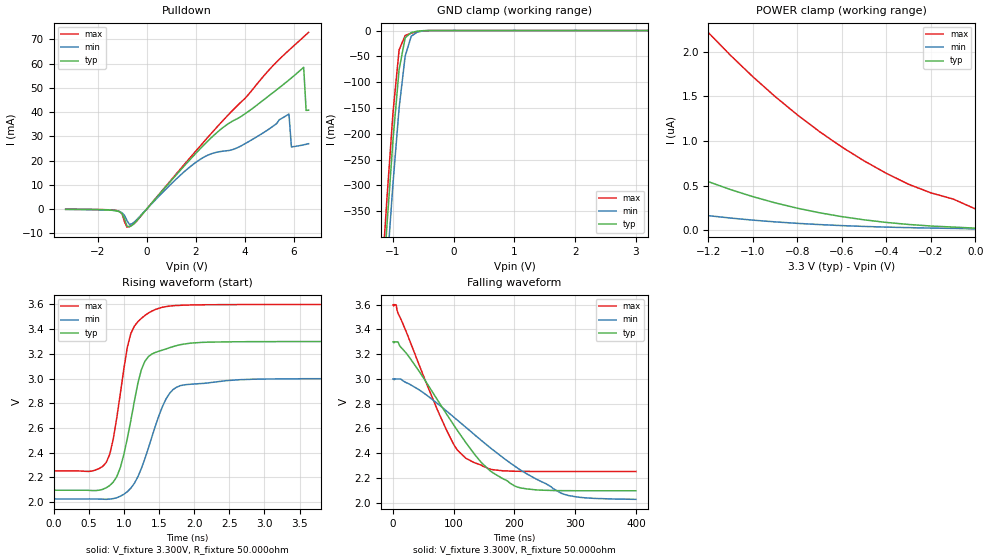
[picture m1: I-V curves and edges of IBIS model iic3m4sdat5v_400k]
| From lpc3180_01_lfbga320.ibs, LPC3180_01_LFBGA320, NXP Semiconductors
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| iic3m4sdat5v
|   IIC Pad
|   Serial Data Signal
| Normal 400 kHz Open-drain Mode (ehs=0)
[Model]   iic3m4sdat5v_400k | of iic3m4sdat5v
Model_type   I/O_open_drain
Polarity   Non-Inverting
|  Reciever Thresholds
Vinl   = 0.99V
Vinh   = 2.31V
| AC Test Load Conditions
Vref   = 0
Cref   = 0
Rref   = 1000000000
Vmeas   = 1.65
| [Process Range]   typical   min   max
| C_comp edge width   400.000ps   400.000ps   400.000ps
| C_comp Tstrobe   40.000fs   40.000fs   40.000fs
C_comp   1.627pF   1.571pF   1.694pF
[Temperature Range]   25   125   -40
[Voltage Range]   3.30V   3.00V   3.60V
[GND Clamp Reference]   0.00V   0.00V   0.00V
[Pulldown Reference]   0.00V   0.00V   0.00V
[POWER Clamp Reference]   3.30V   3.00V   3.60V
[Pullup Reference]   3.30V   3.00V   3.60V
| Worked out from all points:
|   slope of the pulldown table from 0 to 0.495 V, typ, clamps not added: 84.6 ohm
|   GND clamp passes 1 mA (typ) near -0.57 V on its own axis
|   rising waveform, V_fixture 3.300V, R_fixture 50.000ohm: 20-80 % time 266ps typ, 364ps min, 231ps max; typ from 2.1 V to 3.3 V
|   falling waveform, V_fixture 3.300V, R_fixture 50.000ohm: 20-80 % time 100ns typ, 152ns min, 68.8ns max; typ from 3.3 V to 2.1 V
[GND Clamp]
| ref voltage   0.00V   0.00V   0.00V
|   Voltage   I(typ)   I(min)   I(max)
-3.3V     -4.643A    -4.695A    -4.614A
-1.2V     -555.7mA   -637.3mA   -505.9mA
-1.1V     -377.4mA   -461.5mA   -325.3mA
-1V       -211.1mA   -295.8mA   -158.4mA
-900mV    -75.75mA   -150.4mA   -37.68mA
-800mV    -14.14mA   -49.49mA   -9.569mA
-700mV    -4.026mA   -11.01mA   -5.191mA
-600mV    -1.318mA   -2.976mA   -2.281mA
-500mV    -260.9uA   -616.2uA   -536.9uA
3.2V      14.3nA     24.62nA    32.14nA
[Power Clamp]   | Vtable = Vcc - Vpad
| ref voltage   3.30V   3.00V   3.60V
|   Voltage   I(typ)   I(min)   I(max)
-3.3V     5.245uA    2.002uA    29.68uA
-3.1V     4.436uA    1.702uA    22.91uA
-2.8V     3.477uA    1.307uA    15.06uA
-2.3V     2.236uA    785.6nA    7.494uA
-2V       1.641uA    549.3nA    5.219uA
-1.7V     1.148uA    366nA      3.8uA
-1.5V     874.4nA    270.7nA    3.094uA
-1.2V     544.7nA    163.9nA    2.215uA
-900mV    307.4nA    93.98nA    1.498uA
-600mV    152.7nA    52.35nA    932.3nA
-300mV    65.03nA    29.37nA    514.9nA
0V        23.89nA    15.31nA    238.6nA
[Pulldown]
| ref voltage   0.00V   0.00V   0.00V
|   Voltage   I(typ)   I(min)   I(max)
-3.3V     -95.96uA   -104.1uA   -74.67uA
-1.2V     -777.2uA   -758uA     -659.6uA
-1V       -1.884mA   -1.532mA   -1.944mA
-800mV    -7.105mA   -4.771mA   -7.441mA
-500mV    -5.866mA   -5.302mA   -5.87mA
2.1V      24.01mA    19.96mA    25.04mA
3.8V      37.91mA    25.82mA    43.69mA
5.8V      53.26mA    39.21mA    65.53mA
5.9V      54.1mA     25.66mA    66.46mA
6.4V      58.48mA    26.5mA     71.05mA
6.5V      40.69mA    26.73mA    71.98mA
6.6V      40.8mA     26.97mA    72.91mA
[Ramp]
R_load   = 50.000ohm
|   dV/dt(typ)   dV/dt(min)   dV/dt(max)
dV/dt_r   722.648mV/270.000ps   584.921mV/360.000ps   808.935mV/230.000ps
dV/dt_f   67.293mV/11.230ns   22.123mV/7.070ns   155.055mV/13.800ns
[Rising Waveform]  | cubic spline decimation from 2001 points
V_fixture   = 3.300V
V_fixture_min = 3.000V
V_fixture_max = 3.600V
R_fixture   = 50.000ohm
|   Time   V(typ)   V(min)   V(max)
0s        2.096V     2.025V     2.252V
650ps     2.096V     2.024V     2.272V
850ps     2.162V     2.028V     2.512V
1.05ns    2.517V     2.084V     3.255V
1.15ns    2.817V     2.152V     3.425V
1.25ns    3.073V     2.273V     3.488V
1.35ns    3.178V     2.439V     3.531V
1.6ns     3.24V      2.835V     3.583V
1.85ns    3.279V     2.948V     3.595V
100ns     3.3V       3V         3.6V
[Falling Waveform]  | cubic spline decimation from 40001 points
V_fixture   = 3.300V
V_fixture_min = 3.000V
V_fixture_max = 3.600V
R_fixture   = 50.000ohm
|   Time   V(typ)   V(min)   V(max)
0s        3.3V       3V         3.6V
5.16ns    3.3V       3V         3.599V
43.18ns   3.061V     2.912V     3.111V
88.28ns   2.715V     2.74V      2.585V
103.5ns   2.602V     2.677V     2.443V
119.7ns   2.487V     2.61V      2.36V
159.1ns   2.261V     2.448V     2.272V
206.4ns   2.124V     2.275V     2.254V
289.6ns   2.097V     2.057V     2.252V
400ns     2.096V     2.027V     2.252V
